DATA_BLOCK "DB_WARNING"
TITLE =
{ S7_language := '9(1) Inglese (Stati Uniti)  09.12.2014  12:08:08' }
VERSION : 0.1


  STRUCT
   D25_Q01 : BOOL ;	//S.T. CONDIZIONATORE
   D25_F01 : BOOL ;	//TEMPERATURA ALTA ARMADIO ELETTRICO
   E54_Q01 : BOOL ;	//S.T. GRU ORIENTABILE
   E54_XY28_0 : BOOL ;	//GRU ORIENTABILE FUORI POSIZIONE
   E09_S01_HH : BOOL ;	//ALTISSIMO LIVELLO OLIO CENTRALINA IDRAULICA
   E09_S01_H : BOOL ;	//ALTO LIVELLO OLIO CENTRALINA IDRAULICA
   E09_S01_L : BOOL ;	//BASSO LIVELLO OLIO CENTRALINA IDRAULICA
   E09_S01_LL : BOOL ;	//BASSISSIMO LIVELLO OLIO CENTRALINA IDRAULICA
   E51_T01 : BOOL ;	//ALTA CORRENTE MOTORE FRESATRICE PLANETARIA 1
   E52_T01 : BOOL ;	//ALTA CORRENTE MOTORE FRESATRICE PLANETARIA 2
   E61_S11_1 : BOOL ;	//BASSO LIVELLO OLIO LUBRIFICAZIONE 1
   E62_S17_1 : BOOL ;	//BASSO LIVELLO OLIO LUBRIFICAZIONE 2 WG1
   E62_S17_4 : BOOL ;	//BASSO LIVELLO OLIO LUBRIFICAZIONE 2 WG2
   E63_B11_4 : BOOL ;	//BASSO LIVELLO OLIO LUBRIFICAZIONE 3
   E08_S02_3 : BOOL ;	//MANCATA PARTENZA EVACUATORE TRUCIOLI 1
   E08_S28_6 : BOOL ;	//MANCATA PARTENZA EVACUATORE TRUCIOLI 2
   E08_S28_7 : BOOL ;	//MANCATA PARTENZA EVACUATORE TRUCIOLI 3
   E61_S11_11 : BOOL ;	//BASSO LIVELLO OLIO LUBRIFICAZIONE 1
   E61_F20_0 : BOOL ;	//MANCANZA PRESSIONE LUBRIFICAZIONE CONTROPUNTA 1
   E61_F20_1 : BOOL ;	//MANCANZA PRESSIONE LUBRIFICAZIONE GUIDA CONTROPUNTA 1
   E61_F20_2 : BOOL ;	//MANCANZA PRESSIONE LUBRIFICAZIONE SLITTA A CROCE 1
   E61_F20_3 : BOOL ;	//MANCANZA PRESSIONE LUBRIFICAZIONE GUIDA FRESATRICE 1
   E61_F20_4 : BOOL ;	//MANCANZA PRESSIONE LUBRIFICAZIONE FRESATRICE 1
   E61_F21_2 : BOOL ;	//MANCANZA PRESSIONE LUBRIFICAZIONE SERRAGGIO SUPPLEMENTARE 1
   E61_F20_5 : BOOL ;	//MANCANZA PRESSIONE LUBRIFICAZIONE CONTROPUNTA 2
   E61_F20_6 : BOOL ;	//MANCANZA PRESSIONE LUBRIFICAZIONE GUIDA CONTROPUNTA 2
   E61_F20_7 : BOOL ;	//MANCANZA PRESSIONE LUBRIFICAZIONE SLITTA A CROCE 2
   E61_F21_0 : BOOL ;	//MANCANZA PRESSIONE LUBRIFICAZIONE GUIDA FRESATRICE 2
   E61_F21_1 : BOOL ;	//MANCANZA PRESSIONE LUBRIFICAZIONE FRESATRICE 2
   E62_F17_6 : BOOL ;	//INTASAMENTO FILTRO OLIO LUBRIFICAZIONE 2 WG1
   E62_F17_0 : BOOL ;	//MANCANZA PRESSIONE LUBRIFICAZIONE 2 WG1
   E62_S17_1_1 : BOOL ;	//BASSO LIVELLO OLIO LUBRIFICAZIONE 2 WG1
   E62_F17_7 : BOOL ;	//INTASAMENTO FILTRO OLIO LUBRIFICAZIONE 2 WG2
   E62_F17_3 : BOOL ;	//MANCANZA PRESSIONE LUBRIFICAZIONE 2 WG2
   E62_S17_4_1 : BOOL ;	//BASSO LIVELLO OLIO LUBRIFICAZIONE 2 WG2
   E63_B11_41 : BOOL ;	//BASSO LIVELLO OLIO LUBRIFICAZIONE 3
   E63_F21_4 : BOOL ;	//MANCANZA LUBRIFICAZIONE 3 RIDOTTA MONTANTE 1
   E63_F21_5 : BOOL ;	//MANCANZA LUBRIFICAZIONE 3 MONTANTE 1
   E63_F21_6 : BOOL ;	//MANCANZA LUBRIFICAZIONE 3 RIDOTTA MONTANTE 2
   E63_F21_7 : BOOL ;	//MANCANZA LUBRIFICAZIONE 3 MONTANTE 2
   G76_F28_5 : BOOL ;	//MANCANZA PEZZO SU MANDRINO
   SPARE1 : BOOL ;
   SPARE2 : BOOL ;
   SPARE3 : BOOL ;
   SPARE4 : BOOL ;
   SPARE5 : BOOL ;
   SPARE6 : BOOL ;
   SPARE7 : BOOL ;
   SPARE8 : BOOL ;
   SPARE9 : BOOL ;
   SPARE10 : BOOL ;
   SPARE11 : BOOL ;
   SPARE12 : BOOL ;
   SPARE13 : BOOL ;
   SPARE14 : BOOL ;
   SPARE15 : BOOL ;
   SPARE16 : BOOL ;
   SPARE17 : BOOL ;
   SPARE18 : BOOL ;
   SPARE19 : BOOL ;
   SPARE20 : BOOL ;
   SPARE21 : BOOL ;
   SPARE22 : BOOL ;
   SPARE23 : BOOL ;
  END_STRUCT ;
BEGIN
   D25_Q01 := FALSE;
   D25_F01 := FALSE;
   E54_Q01 := FALSE;
   E54_XY28_0 := FALSE;
   E09_S01_HH := FALSE;
   E09_S01_H := FALSE;
   E09_S01_L := FALSE;
   E09_S01_LL := FALSE;
   E51_T01 := FALSE;
   E52_T01 := FALSE;
   E61_S11_1 := FALSE;
   E62_S17_1 := FALSE;
   E62_S17_4 := FALSE;
   E63_B11_4 := FALSE;
   E08_S02_3 := FALSE;
   E08_S28_6 := FALSE;
   E08_S28_7 := FALSE;
   E61_S11_11 := FALSE;
   E61_F20_0 := FALSE;
   E61_F20_1 := FALSE;
   E61_F20_2 := FALSE;
   E61_F20_3 := FALSE;
   E61_F20_4 := FALSE;
   E61_F21_2 := FALSE;
   E61_F20_5 := FALSE;
   E61_F20_6 := FALSE;
   E61_F20_7 := FALSE;
   E61_F21_0 := FALSE;
   E61_F21_1 := FALSE;
   E62_F17_6 := FALSE;
   E62_F17_0 := FALSE;
   E62_S17_1_1 := FALSE;
   E62_F17_7 := FALSE;
   E62_F17_3 := FALSE;
   E62_S17_4_1 := FALSE;
   E63_B11_41 := FALSE;
   E63_F21_4 := FALSE;
   E63_F21_5 := FALSE;
   E63_F21_6 := FALSE;
   E63_F21_7 := FALSE;
   G76_F28_5 := FALSE;
   SPARE1 := FALSE;
   SPARE2 := FALSE;
   SPARE3 := FALSE;
   SPARE4 := FALSE;
   SPARE5 := FALSE;
   SPARE6 := FALSE;
   SPARE7 := FALSE;
   SPARE8 := FALSE;
   SPARE9 := FALSE;
   SPARE10 := FALSE;
   SPARE11 := FALSE;
   SPARE12 := FALSE;
   SPARE13 := FALSE;
   SPARE14 := FALSE;
   SPARE15 := FALSE;
   SPARE16 := FALSE;
   SPARE17 := FALSE;
   SPARE18 := FALSE;
   SPARE19 := FALSE;
   SPARE20 := FALSE;
   SPARE21 := FALSE;
   SPARE22 := FALSE;
   SPARE23 := FALSE;
END_DATA_BLOCK

